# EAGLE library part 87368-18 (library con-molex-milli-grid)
RECEPTACAL
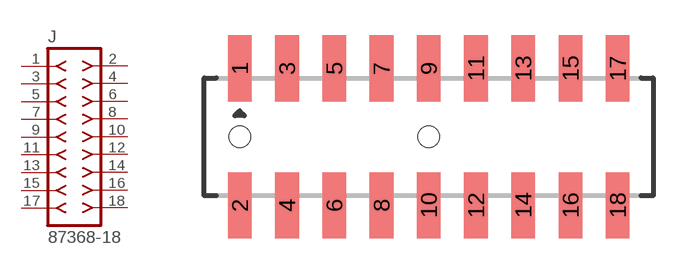
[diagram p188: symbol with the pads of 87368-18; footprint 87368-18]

Designator prefix J

## 87368-18  [87368-18]
1  1  pas
2  2  pas
3  3  pas
4  4  pas
5  5  pas
6  6  pas
7  7  pas
8  8  pas
9  9  pas
10  10  pas
11  11  pas
12  12  pas
13  13  pas
14  14  pas
15  15  pas
16  16  pas
17  17  pas
18  18  pas

## Footprint 87368-18 (pad centres in mm)
RECEPTACAL SMD Dual Row, Side Entry
smd 1 x 2.8: 1 -8,2.9; 2 -8,-2.9; 3 -6,2.9; 4 -6,-2.9; 5 -4,2.9; 6 -4,-2.9; 7 -2,2.9; 8 -2,-2.9; 9 0,2.9; 10 0,-2.9; 11 2,2.9; 12 2,-2.9; 13 4,2.9; 14 4,-2.9; 15 6,2.9; 16 6,-2.9; 17 8,2.9; 18 8,-2.9
hole 0.914 at -8,0
hole 0.914 at 0,0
